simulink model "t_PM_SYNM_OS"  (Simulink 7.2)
settings: Solver=ode3  StartTime=0.0  StopTime=0.5  FixedStep=10e-6  MaxStep=1e-4  RelTol=1e-4  AbsTol=1e-4
libraries: simulink x1

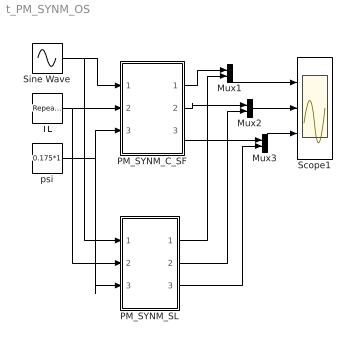
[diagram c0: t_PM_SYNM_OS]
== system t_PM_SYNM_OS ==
  Mux1 : Mux  Inputs=2
  Mux2 : Mux  Inputs=2
  Mux3 : Mux  Inputs=2
  PM_SYNM_C_SF : Subsystem  mask(PSM-C-S-Function Block){R1=2.875, Lq=8.5e-3, Ld=8.5e-3, P=8, J=0.8e-3, D=0.5e-3, W0=0}
      mask prompts: R1 "Stator Resistance"; Lq "Q-Axis Inductance"; Ld "D-Axis Inductance"; P "Number of Poles"; J "Moment of Inertia"; D "Damping Coefficient"; W0 "initial ang. speed"
      mask help: Open source Permanent Magnet SYNCHRON MOTOR modeled as Simulink C-S-Function Blocks Input Vector u: u[0,1,2]= Three phase stator Voltages u[3]= Load Torque u[4]= PSI Output Vector y: y[0,1,2]= Three phase stator Currents y[3]= Te y[4]= Ang. Velocity W Parameter Vector p: p[0]= R1 p[1]= Lq p[2]= Ld p[3]= Number of Poles P p[4]= Moment of Inertia J p[5]= Damp. Coef. D p[6]= Initial Ang. Velocity W0 You can pause the simulation during running, change the Parameters you want and continue the Simulation
  PM_SYNM_SL : Subsystem  mask(PSM-SL){R1=2.875, Lq=8.5e-3, Ld=8.5e-3, P=8, J=0.8e-3, D=0.5e-3, omm0=0}
      mask prompts: R1 "Stator Resistance"; Lq "Q-Axis Inductance"; Ld "D-Axis Inductance"; P "Number of Poles"; J "Moment of Inertia"; D "Damping Coefficient"; omm0 "initial ang. speed"
      mask help: Open source Permanent Magnet SYNCHRON MOTOR modeled in Simulink Blocks Input Vector u: u[0,1,2]= Three phase stator Voltages u[3]= Load Torque u[4]= PSI Output Vector y: y[0,1,2]= Three phase stator Currents y[3]= Te y[4]= Ang. Velocity W Parameter Vector p: p[0]= R1 p[1]= Lq p[2]= Ld p[3]= Number of Poles P p[4]= Moment of Inertia J p[5]= Damp. Coef. D p[6]= Initial Ang. Velocity W0 You can pause the simulation during running, change the Parameters you want and continue the Simulation
  Scope1 : Scope  NumInputPorts=3
  Sine Wave : Sin  Amplitude=230*sqrt(2)  Frequency=50*2*pi  Phase=[0, -2*pi/3, -4*pi/3]  SampleTime=0
  TL : simulink/Sources/Repeating Sequence  SystemSampleTime=-1  rep_seq_t="[0      0.15     0.1501   0.3     0.301   1]"  rep_seq_y="[0        0             1         1         -1      -1]*20"
  psi : Constant  Value=0.175*1
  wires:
  Sine Wave/1 -> PM_SYNM_C_SF/1(Vabc), PM_SYNM_SL/1(Vabc)
  TL/1 -> PM_SYNM_C_SF/2(TL), PM_SYNM_SL/2(TL)
  Mux1/1 -> Scope1/1
  Mux2/1 -> Scope1/2
  Mux3/1 -> Scope1/3
  PM_SYNM_C_SF/1(Iabc) -> Mux1/1
  PM_SYNM_C_SF/2(TE) -> Mux2/1
  psi/1 -> PM_SYNM_C_SF/3(PSI), PM_SYNM_SL/3(PSI)
  PM_SYNM_SL/2(Te) -> Mux2/2
  PM_SYNM_SL/1(Iabc) -> Mux1/2
  PM_SYNM_SL/3(Wm) -> Mux3/2
  PM_SYNM_C_SF/3(Wm) -> Mux3/1

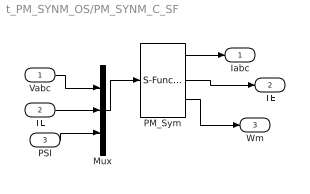
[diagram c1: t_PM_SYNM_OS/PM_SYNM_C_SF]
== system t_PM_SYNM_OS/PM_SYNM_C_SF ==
  Vabc : Inport  OutDataType=sfix(16)  OutScaling=2^0
  TL : Inport  Port=2  OutDataType=sfix(16)  OutScaling=2^0
  PSI : Inport  Port=3  OutDataType=sfix(16)  OutScaling=2^0
  Mux : Mux  Inputs=[3 1 1]
  PM_Sym : S-Function  FunctionName=s_PM_Synm_OS  Parameters=[R1 Lq Ld P J D W0]  EnableBusSupport=off
  Iabc : Outport  OutDataType=sfix(16)  OutScaling=2^0
  TE : Outport  Port=2  OutDataType=sfix(16)  OutScaling=2^0
  Wm : Outport  Port=3  OutDataType=sfix(16)  OutScaling=2^0
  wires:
  PM_Sym/1 -> Iabc/1
  PM_Sym/2 -> TE/1
  PM_Sym/3 -> Wm/1
  Mux/1 -> PM_Sym/1
  Vabc/1 -> Mux/1
  TL/1 -> Mux/2
  PSI/1 -> Mux/3

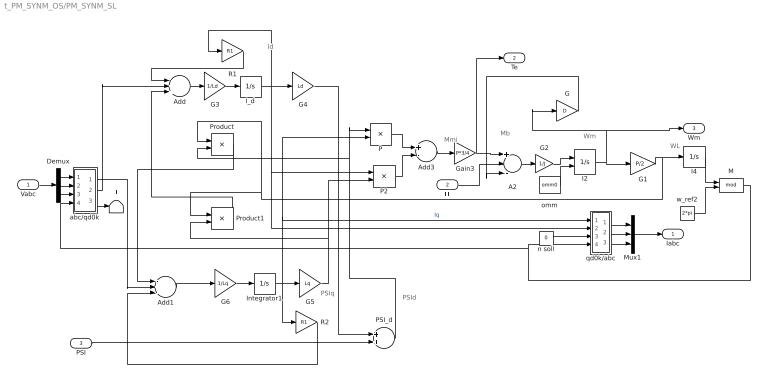
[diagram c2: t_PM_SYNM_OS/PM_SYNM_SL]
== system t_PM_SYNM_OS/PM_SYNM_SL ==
  note: PSId
  note: Id
  note: PSIq
  note: WL
  note: Wm
  note: Mmi
  note: Mb
  Vabc : Inport
  TL : Inport  Port=2
  PSI : Inport  Port=3
  A2 : Sum  Inputs=+--
  Add : Sum  Inputs=-++
  Add1 : Sum  Inputs=-+-
  Add3 : Sum  Inputs=+-
  Demux : Demux  Outputs=3
  G : Gain  Gain=D
  G1 : Gain  Gain=P/2
  G2 : Gain  Gain=1/J
  G3 : Gain  Gain=1/Ld
  G4 : Gain  Gain=Ld
  G5 : Gain  Gain=Lq
  G6 : Gain  Gain=1/Lq
  Gain3 : Gain  Gain=P*3/4
  I2 : Integrator  InitialConditionSource=external
  I4 : Integrator
  I_d : Integrator
  Integrator1 : Integrator
  M : Math  Operator=mod
  Mux1 : Mux  Inputs=3
  P : Product
  P2 : Product
  PSI_d : Sum
  Product : Product
  Product1 : Product
  R1 : Gain  Gain=R1
  R2 : Gain  Gain=R1
  T : Terminator
  abc/qd0k : Subsystem
  n soll : Constant  Value=0
  omm : Constant  Value=omm0
  qd0k/abc : Subsystem
  w_ref2 : Constant  Value=2*pi
  Iabc : Outport
  Te : Outport  Port=2
  Wm : Outport  Port=3
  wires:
  G6/1 -> Integrator1/1
  G3/1 -> I_d/1
  Mux1/1 -> Iabc/1
  qd0k/abc/3(c) -> Mux1/3
  qd0k/abc/1(a) -> Mux1/1
  qd0k/abc/2(b) -> Mux1/2
  Demux/3 -> abc/qd0k/3(c)
  Demux/1 -> abc/qd0k/1(a)
  Demux/2 -> abc/qd0k/2(b)
  Vabc/1 -> Demux/1
  PSI/1 -> PSI_d/2
  G1/1 -> I4/1, Product/1, Product1/1
  G5/1 -> Product1/2, P2/2
  PSI_d/1 -> Product/2, P/1
  G4/1 -> PSI_d/1
  n soll/1 -> qd0k/abc/3(0k)
  abc/qd0k/3(0k) -> T/1
  R1/1 -> Add/1
  R2/1 -> Add1/3
  A2/1 -> G2/1
  G2/1 -> I2/1
  I2/1 -> G1/1, Wm/1, G/1
  Product/1 -> Add1/1
  Product1/1 -> Add/3
  Gain3/1 -> A2/1, Te/1
  Add3/1 -> Gain3/1
  P/1 -> Add3/1
  P2/1 -> Add3/2
  abc/qd0k/1(qk) -> Add1/2
  I_d/1 -> G4/1, P2/1, qd0k/abc/2(dk), R1/1
  Add/1 -> G3/1
  Integrator1/1 -> G5/1, P/2, qd0k/abc/1(qk), R2/1  "Iq"
  Add1/1 -> G6/1
  I4/1 -> M/1
  TL/1 -> A2/2
  w_ref2/1 -> M/2
  M/1 -> abc/qd0k/4(th), qd0k/abc/4(th)
  abc/qd0k/2(dk) -> Add/2
  omm/1 -> I2/2
  G/1 -> A2/3

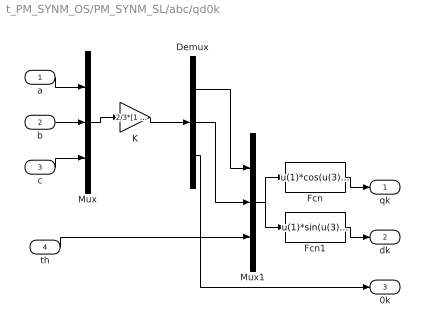
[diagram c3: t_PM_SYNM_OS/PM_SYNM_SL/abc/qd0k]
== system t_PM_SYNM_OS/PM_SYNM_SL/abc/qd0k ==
  a : Inport  OutDataType=sfix(16)  OutScaling=2^0
  b : Inport  Port=2  OutDataType=sfix(16)  OutScaling=2^0
  c : Inport  Port=3  OutDataType=sfix(16)  OutScaling=2^0
  th : Inport  Port=4  OutDataType=sfix(16)  OutScaling=2^0
  Demux : Demux  Outputs=3
  Fcn : Fcn  Expr=u(1)*cos(u(3)) - u(2)*sin(u(3))
  Fcn1 : Fcn  Expr=u(1)*sin(u(3)) + u(2)*cos(u(3))
  K : Gain  Gain="2/3*[1   -.5   -.5;  0   -sqrt(3)/2   sqrt(3)/2;  .5    .5    .5]"  Multiplication=Matrix(K*u)  ParameterDataType=sfix(16)  ParameterScaling=2^0  OutDataType=sfix(16)  OutScaling=2^0
  Mux : Mux  Inputs=3
  Mux1 : Mux  Inputs=3
  qk : Outport
  dk : Outport  Port=2
  0k : Outport  Port=3
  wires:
  c/1 -> Mux/3
  b/1 -> Mux/2
  K/1 -> Demux/1
  Mux/1 -> K/1
  a/1 -> Mux/1
  Mux1/1 -> Fcn1/1, Fcn/1
  Fcn/1 -> qk/1
  Fcn1/1 -> dk/1
  th/1 -> Mux1/3
  Demux/3 -> 0k/1
  Demux/1 -> Mux1/1
  Demux/2 -> Mux1/2

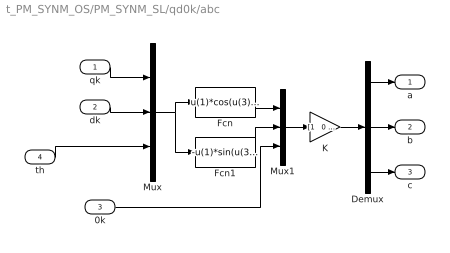
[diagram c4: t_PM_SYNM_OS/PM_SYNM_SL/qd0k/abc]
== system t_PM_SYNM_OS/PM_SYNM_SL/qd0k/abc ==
  qk : Inport  OutDataType=sfix(16)  OutScaling=2^0
  dk : Inport  Port=2  OutDataType=sfix(16)  OutScaling=2^0
  0k : Inport  Port=3  OutDataType=sfix(16)  OutScaling=2^0
  th : Inport  Port=4  OutDataType=sfix(16)  OutScaling=2^0
  Demux : Demux  Outputs=3
  Fcn : Fcn  Expr=u(1)*cos(u(3)) + u(2)*sin(u(3))
  Fcn1 : Fcn  Expr=-u(1)*sin(u(3)) + u(2)*cos(u(3))
  K : Gain  Gain="[1   0  1 ;  -.5   -sqrt(3)/2    1 ;  -.5    sqrt(3)/2    1]"  Multiplication=Matrix(K*u)  ParameterDataType=sfix(16)  ParameterScaling=2^0  OutDataType=sfix(16)  OutScaling=2^0
  Mux : Mux  Inputs=3
  Mux1 : Mux  Inputs=3
  a : Outport
  b : Outport  Port=2
  c : Outport  Port=3
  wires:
  qk/1 -> Mux/1
  dk/1 -> Mux/2
  Mux/1 -> Fcn/1, Fcn1/1
  K/1 -> Demux/1
  Mux1/1 -> K/1
  Fcn/1 -> Mux1/1
  Fcn1/1 -> Mux1/2
  Demux/1 -> a/1
  Demux/2 -> b/1
  Demux/3 -> c/1
  th/1 -> Mux/3
  0k/1 -> Mux1/3
